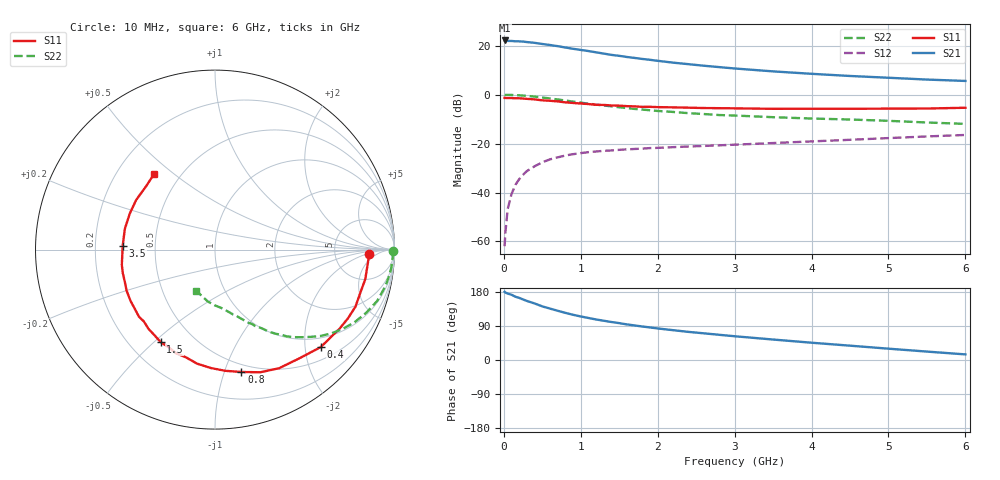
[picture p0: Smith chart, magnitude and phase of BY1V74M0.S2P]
! SIEMENS Small Signal Semiconductors
! BFY420
! Si NPN RF SIEGET Grounded Emitter Transistor in MICRO-X
! VCE = 1.75 V  IC = 4 mA
! Common Emitter S-Parameters:  October  1996
# GHz  S  MA  R  50
!  f  S11  S21  S12  S22
! GHz  MAG  ANG  MAG  ANG  MAG  ANG  MAG  ANG
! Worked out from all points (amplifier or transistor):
!   36 points, 10 MHz to 6 GHz, reference 50 ohm
!   highest |S21| = 22.2 dB at 10 MHz (marker M1)
!   |S21| within 3 dB of that: start of sweep to 821.7 MHz
!   unconditionally stable (mu >= 1): 3.331 GHz to end of sweep
!   at 250 MHz: K = 0.10, MSG = 27.2 dB, |S12| = -32.7 dB
!   at 1.4 GHz: K = 0.47, MSG = 19.5 dB, |S12| = -22.8 dB
!   at 6 GHz: K = 1.17, MAG = 8.6 dB, |S12| = -16.5 dB
!   S11 on the Smith chart (normalised r, x): 10 MHz: 13, -2; 400 MHz: 0.77, -2.34; 800 MHz: 0.43, -1.14; 1.5 GHz: 0.33, -0.52; 3.5 GHz: 0.32, +0.02; 6 GHz: 0.36, +0.43
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0.01  0.8593 -1.5  12.85 180.0  0.0008 104.2  0.9919 -0.6
0.02  0.8583 -2.4  12.81 177.9  0.0015 79.8  0.9904 -1.1
0.05  0.8544 -5.6  12.57 175.3  0.0046 85.9  0.9907 -3.0
0.1  0.8533 -11.2  12.54 172.2  0.0093 82.4  0.9872 -6.0
0.15  0.8446 -16.5  12.37 167.0  0.0143 80.3  0.9796 -9.0
0.25  0.834 -27.3  12.19 159.7  0.0231 74.7  0.959 -14.7
0.4  0.8012 -42.7  11.49 149.2  0.0344 67.5  0.913 -22.7
0.5  0.7668 -52.2  10.88 141.5  0.0414 62.9  0.8757 -27.6
0.6  0.7512 -61.6  10.38 135.7  0.0477 58.5  0.837 -31.9
0.7  0.7286 -69.7  9.829 129.9  0.0523 54.8  0.7985 -35.8
0.8  0.6977 -77.8  9.215 124.4  0.0571 50.6  0.7598 -39.3
0.9  0.6777 -85.2  8.684 119.3  0.0608 48.1  0.7223 -42.3
1.1  0.6433 -98.9  7.805 110.9  0.0669 43.6  0.6564 -48.0
1.3  0.6171 -110.5  6.921 103.6  0.0712 39.9  0.6 -52.2
1.5  0.5974 -120.5  6.229 97.3  0.0746 37.3  0.5537 -56.1
1.8  0.5634 -134.7  5.381 88.4  0.079 34.4  0.4958 -60.6
2.2  0.5505 -148.8  4.521 78.7  0.0846 31.6  0.4442 -65.9
2.8  0.53 -165.9  3.665 66.5  0.0922 29.6  0.3838 -72.5
3.5  0.5146 177.5  2.997 54.0  0.1027 27.7  0.3469 -79.2
4.5  0.5155 157.0  2.414 37.8  0.1196 24.5  0.311 -90.1
5.5  0.5215 137.4  2.039 22.2  0.1401 20.0  0.2701 -105.1
6  0.5405 129.0  1.91 14.8  0.1503 17.2  0.2528 -114.4
